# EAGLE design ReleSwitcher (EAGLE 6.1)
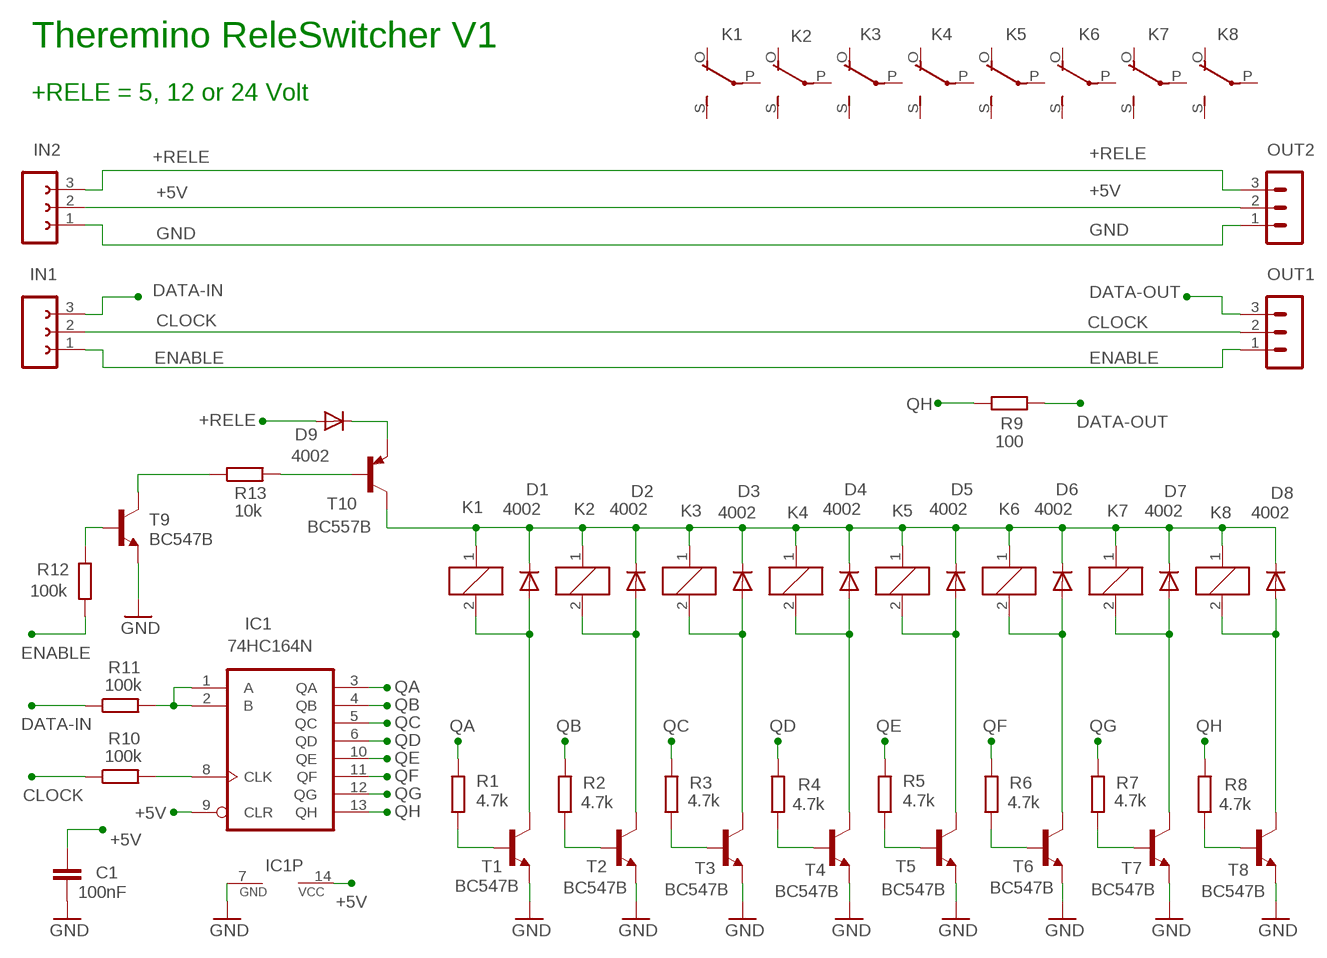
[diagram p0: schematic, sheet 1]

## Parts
C1  100nF  C-EU025-024X044  [C025-024X044]
D1  4002  DIODE-DO34-7  [DO34-7]
D2  4002  DIODE-DO34-7  [DO34-7]
D3  4002  DIODE-DO34-7  [DO34-7]
D4  4002  DIODE-DO34-7  [DO34-7]
D5  4002  DIODE-DO34-7  [DO34-7]
D6  4002  DIODE-DO34-7  [DO34-7]
D7  4002  DIODE-DO34-7  [DO34-7]
D8  4002  DIODE-DO34-7  [DO34-7]
D9  4002  DIODE-DO34-7  [DO34-7]
IC1  74HC164N  [DIL14]
IN1  FE03-1"  [FE03-1]
IN2  FE03-1"  [FE03-1]
K1  E3206S  [E3206S]
K2  E3206S  [E3206S]
K3  E3206S  [E3206S]
K4  E3206S  [E3206S]
K5  E3206S  [E3206S]
K6  E3206S  [E3206S]
K7  E3206S  [E3206S]
K8  E3206S  [E3206S]
OUT1  MA03-1N  [MA03-1]
OUT2  MA03-1N  [MA03-1]
R1  4.7k  R-EU_0204/7  [0204/7]
R2  4.7k  R-EU_0204/7  [0204/7]
R3  4.7k  R-EU_0204/7  [0204/7]
R4  4.7k  R-EU_0204/7  [0204/7]
R5  4.7k  R-EU_0207/10  [0207/10]
R6  4.7k  R-EU_0207/10  [0207/10]
R7  4.7k  R-EU_0207/10  [0207/10]
R8  4.7k  R-EU_0207/10  [0207/10]
R9  100  R-EU_0207/10  [0207/10]
R10  100k  R-EU_0207/15  [0207/15]
R11  100k  R-EU_0207/12  [0207/12]
R12  100k  R-EU_0207/15  [0207/15]
R13  10k  R-EU_0204/7  [0204/7]
T1  BC547B  -NPN-TO92-CBE  [TO92-CBE]
T2  BC547B  -NPN-TO92-CBE  [TO92-CBE]
T3  BC547B  -NPN-TO92-CBE  [TO92-CBE]
T4  BC547B  -NPN-TO92-CBE  [TO92-CBE]
T5  BC547B  -NPN-TO92-CBE  [TO92-CBE]
T6  BC547B  -NPN-TO92-CBE  [TO92-CBE]
T7  BC547B  -NPN-TO92-CBE  [TO92-CBE]
T8  BC547B  -NPN-TO92-CBE  [TO92-CBE]
T9  BC547B  -NPN-TO92-CBE  [TO92-CBE]
T10  BC557B  -PNP-TO92-CBE  [TO92-CBE]

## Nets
+5V: C1.1 IC1.9(CLR) IC1.14(VCC) IN2.2 OUT2.2
+RELE: D9.A IN2.3 OUT2.3
CLOCK: IN1.2 OUT1.2 R10.1
DATA-IN: IN1.3 R11.1
DATA-OUT: OUT1.3 R9.1
ENABLE: IN1.1 OUT1.1 R12.2
GND: C1.2 IC1.7(GND) IN2.1 OUT2.1 T1.E T2.E T3.E T4.E T5.E T6.E T7.E T8.E T9.E
N$1: R4.1 T4.B
N$2: R8.1 T8.B
N$4: R3.1 T3.B
N$5: D1.C D2.C D3.C D4.C D5.C D6.C D7.C D8.C K1.1 K2.1 K3.1 K4.1 K5.1 K6.1 K7.1 K8.1 T10.C
N$6: R2.1 T2.B
N$8: R1.1 T1.B
N$10: D4.A K4.2 T4.C
N$11: D3.A K3.2 T3.C
N$12: D2.A K2.2 T2.C
N$13: D1.A K1.2 T1.C
N$14: R13.1 T9.C
N$15: R13.2 T10.B
N$16: R12.1 T9.B
N$17: IC1.1(A) IC1.2(B) R11.2
N$18: IC1.8(CLK) R10.2
N$19: R7.1 T7.B
N$20: D9.C T10.E
N$22: R6.1 T6.B
N$25: R5.1 T5.B
N$27: D8.A K8.2 T8.C
N$28: D7.A K7.2 T7.C
N$29: D6.A K6.2 T6.C
N$30: D5.A K5.2 T5.C
QA: IC1.3(QA) R1.2
QB: IC1.4(QB) R2.2
QC: IC1.5(QC) R3.2
QD: IC1.6(QD) R4.2
QE: IC1.10(QE) R5.2
QF: IC1.11(QF) R6.2
QG: IC1.12(QG) R7.2
QH: IC1.13(QH) R8.2 R9.2
Unconnected: K1.O(2:O) K1.P(2:P) K1.S(2:S) K2.O(2:O) K2.P(2:P) K2.S(2:S) K3.O(2:O) K3.P(2:P) K3.S(2:S) K4.O(2:O) K4.P(2:P) K4.S(2:S) K5.O(2:O) K5.P(2:P) K5.S(2:S) K6.O(2:O) K6.P(2:P) K6.S(2:S) K7.O(2:O) K7.P(2:P) K7.S(2:S) K8.O(2:O) K8.P(2:P) K8.S(2:S)

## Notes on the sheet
- Theremino ReleSwitcher V1
- +RELE = 5, 12 or 24 Volt

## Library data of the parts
C1 = 00-LIVIO:C-EU: CAPACITOR, European symbol
D1-D9 = 00-LIVIO:DIODE-: DIODE
IC1 = 74xx-eu:74*164: 8-bit parallel out SHIFT REGISTER
IN1 IN2 = 02-con-lsta-F:FE03-1: FEMALE HEADER
K1-K8 = relay:E3206S: RELAY 1 x switch, Eichhoff/distributor Schukat
OUT1 OUT2 = 03-con-lstb-M:MA03-1: PIN HEADER
R1-R13 = 00-LIVIO:R-EU_: RESISTOR, European symbol
T1-T9 = 00-LIVIO:*-NPN-: NPN Transistror
T10 = 00-LIVIO:*-PNP-: PNP Transistror

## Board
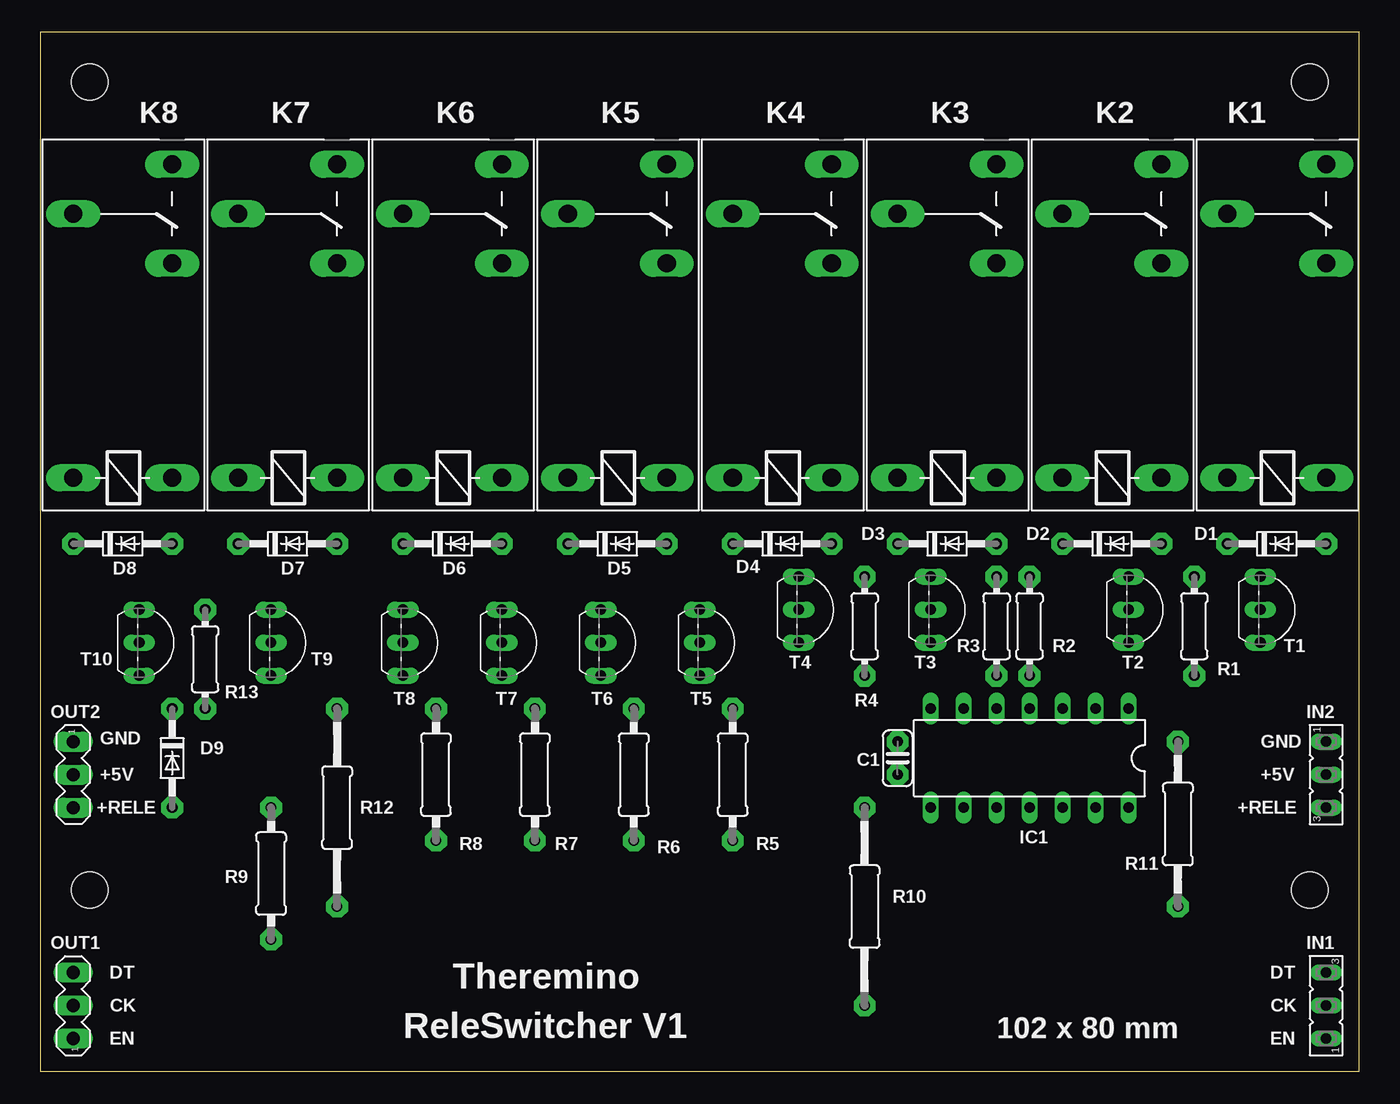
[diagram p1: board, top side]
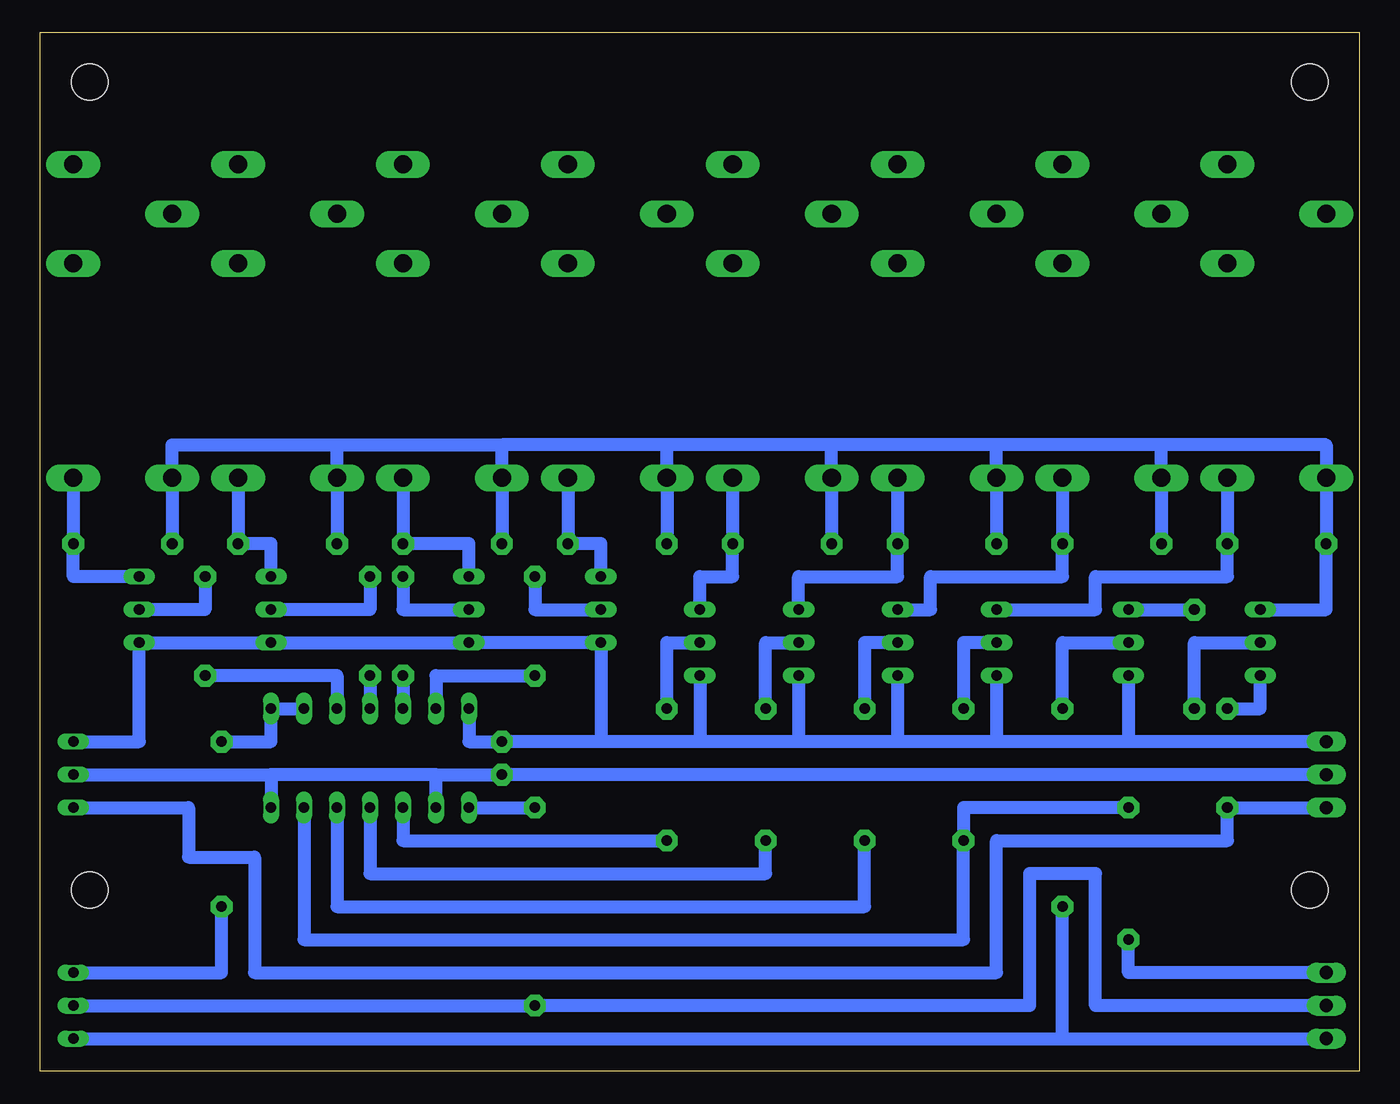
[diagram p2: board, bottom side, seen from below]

Size 101.6 x 80.01 mm. Coordinates in mm from the lower left corner, seen from the top.
Outline: 101.6,80.01 0,80.01 0,0 101.6,0 101.6,80.01
Copper layers (1*16): Top 0.035mm / dielectric 1.5mm / Bottom 0.035mm
Design rules: minimum track width 10mil, minimum drill 31mil, track to track 31mil, track to pad 31mil, pad to pad 31mil, via to via 31mil, smd to smd 31mil, copper to edge 31mil, drill to drill 8mil, minimum pad ring 5mil, minimum via ring 8mil, stop-mask expansion 4mil, vias tented up to drill 0mil, thermal gap 47mil
Holes 2.8 mm at 97.79,76.2 3.81,76.2 3.81,13.97 97.79,13.97

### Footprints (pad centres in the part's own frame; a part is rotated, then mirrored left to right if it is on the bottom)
C025-024X044 = drill 0.813 pad 1.676 octagon: 1 -1.27,0; 2 1.27,0
DO34-7 = drill 0.813 pad 1.676 octagon: A 3.81,0; C -3.81,0
DIL14 = drill 0.813 long: 1 -7.62,-3.81; 2 -5.08,-3.81; 3 -2.54,-3.81; 4 0,-3.81; 5 2.54,-3.81; 6 5.08,-3.81; 7 7.62,-3.81; 8 7.62,3.81; 9 5.08,3.81; 10 2.54,3.81; 11 0,3.81; 12 -2.54,3.81; 13 -5.08,3.81; 14 -7.62,3.81
FE03-1 = drill 0.813 long: 1 -2.54,0; 2 0,0; 3 2.54,0
E3206S = drill 1.397 long: 1 -3.175,3.81; 2 -3.175,-3.81; O 13.335,-3.81; P 17.145,3.81; S 20.955,-3.81
MA03-1 = drill 1.016 long: 1 -2.54,0; 2 0,0; 3 2.54,0
0204/7 = drill 0.813 pad 1.676 octagon: 1 -3.81,0; 2 3.81,0
0207/10 = drill 0.813 pad 1.676 octagon: 1 -5.08,0; 2 5.08,0
0207/15 = drill 0.813 pad 1.676 octagon: 1 -7.62,0; 2 7.62,0
0207/12 = drill 0.813 pad 1.676 octagon: 1 -6.35,0; 2 6.35,0
TO92-CBE = drill 0.813 long: B 0,0; C -2.54,0; E 2.54,0

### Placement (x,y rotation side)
C1  66.04,24.13 90 top
D1  95.25,40.64 0 top
D2  82.55,40.64 0 top
D3  69.85,40.64 0 top
D4  57.15,40.64 0 top
D5  44.45,40.64 0 top
D6  31.75,40.64 0 top
D7  19.05,40.64 0 top
D8  6.35,40.64 0 top
D9  10.16,24.13 270 top
IC1  76.2,24.13 180 top
IN1  99.06,5.08 90 top
IN2  99.06,22.86 270 top
K1  95.25,48.9 90 top
K2  82.55,48.9 90 top
K3  69.85,48.9 90 top
K4  57.15,48.9 90 top
K5  44.45,48.9 90 top
K6  31.75,48.9 90 top
K7  19.05,48.9 90 top
K8  6.35,48.9 90 top
OUT1  2.54,5.08 90 top
OUT2  2.54,22.86 270 top
R1  88.9,34.29 270 top
R2  76.2,34.29 270 top
R3  73.66,34.29 270 top
R4  63.5,34.29 270 top
R5  53.34,22.86 270 top
R6  45.72,22.86 270 top
R7  38.1,22.86 270 top
R8  30.48,22.86 270 top
R9  17.78,15.24 90 top
R10  63.5,12.7 90 top
R11  87.63,19.05 90 top
R12  22.86,20.32 270 top
R13  12.7,31.75 270 top
T1  93.98,35.56 270 top
T2  83.82,35.56 270 top
T3  68.58,35.56 270 top
T4  58.42,35.56 270 top
T5  50.8,33.02 270 top
T6  43.18,33.02 270 top
T7  35.56,33.02 270 top
T8  27.94,33.02 270 top
T9  17.78,33.02 270 top
T10  7.62,33.02 270 top

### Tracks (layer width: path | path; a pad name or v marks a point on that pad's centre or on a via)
+5V
  Bottom 1.016: IC1.9 71.12,22.86 | 71.12,22.86 83.82,22.86 | 83.82,22.86 IC1.14 | 71.12,22.86 C1.1 OUT2.2 | IN2.2 83.82,22.86
+RELE
  Bottom 1.016: IN2.3 90.17,20.32 90.17,16.51 85.09,16.51 85.09,7.62 27.94,7.62 27.94,17.78 10.16,17.78 D9.A OUT2.3
CLOCK
  Bottom 1.016: OUT1.2 20.32,5.08 20.32,15.24 25.4,15.24 25.4,5.08 R10.1 IN1.2
DATA-IN
  Bottom 1.016: IN1.3 87.63,7.62 R11.1
DATA-OUT
  Bottom 1.016: OUT1.3 17.78,7.62 R9.1
ENABLE
  Bottom 1.016: IN1.1 22.86,2.54 | 22.86,2.54 OUT1.1 | 22.86,2.54 R12.2
GND
  Bottom 1.016: IC1.7 68.58,25.4 C1.2 58.42,25.4 | 58.42,25.4 T4.E T3.E T2.E T1.E 93.98,25.4 IN2.1 | 27.94,25.4 35.56,25.4 | 35.56,25.4 43.18,25.4 | 43.18,25.4 50.8,25.4 | 50.8,25.4 58.42,25.4 | T6.E 43.18,25.4 | T5.E 50.8,25.4 | T7.E 35.56,25.4 | T8.E 27.94,25.4 | OUT2.1 17.78,25.4 | 17.78,25.4 27.94,25.4 | T9.E 17.78,25.4
N$1
  Bottom 1.016: R4.1 63.5,35.56 T4.B
N$2
  Bottom 1.016: T8.B 30.48,33.02 R8.1
N$4
  Bottom 1.016: R3.1 73.66,35.56 T3.B
N$5
  Bottom 1.016: D1.C K1.1 91.44,48.26 78.74,48.26 | 15.24,48.26 2.54,48.26 K8.1 D8.C 2.54,35.56 T10.C | 15.24,48.26 27.94,48.26 | 27.94,48.26 40.64,48.26 | 40.64,48.26 53.34,48.26 | 53.34,48.26 66.04,48.26 | 78.74,48.26 K2.1 D2.C | 78.74,48.26 66.04,48.26 | D3.C K3.1 66.04,48.26 | D4.C K4.1 53.34,48.26 | 15.24,48.26 K7.1 D7.C | 27.94,48.26 K6.1 D6.C | 40.64,48.26 K5.1 D5.C
N$6
  Bottom 1.016: R2.1 76.2,35.56 T2.B
N$8
  Bottom 1.016: R1.1 88.9,35.56 T1.B
N$10
  Bottom 1.016: K4.2 D4.A 58.42,40.64 T4.C
N$11
  Bottom 1.016: K3.2 D3.A 68.58,40.64 T3.C
N$12
  Bottom 1.016: K2.2 D2.A 83.82,40.64 T2.C
N$13
  Bottom 1.016: K1.2 D1.A 99.06,38.1 T1.C
N$14
  Bottom 1.016: T9.C R13.1
N$15
  Bottom 1.016: R13.2 12.7,33.02 T10.B
N$16
  Bottom 1.016: R12.1 22.86,33.02 T9.B
N$17
  Bottom 1.016: IC1.2 IC1.1 83.82,25.4 R11.2
N$18
  Bottom 1.016: IC1.8 R10.2
N$19
  Bottom 1.016: T7.B 38.1,33.02 R7.1
N$20
  Bottom 1.016: D9.C 7.62,27.94 T10.E
N$22
  Bottom 1.016: R6.1 45.72,33.02 T6.B
N$25
  Bottom 1.016: R5.1 53.34,33.02 T5.B
N$27
  Bottom 1.016: K8.2 D8.A 10.16,38.1 20.32,38.1 20.32,35.56 T8.C
N$28
  Bottom 1.016: K7.2 D7.A 22.86,38.1 33.02,38.1 33.02,35.56 T7.C
N$29
  Bottom 1.016: K6.2 D6.A 35.56,38.1 43.18,38.1 T6.C
N$30
  Bottom 1.016: K5.2 D5.A 48.26,38.1 50.8,38.1 T5.C
QA
  Bottom 1.016: R1.2 78.74,30.48 IC1.3
QB
  Bottom 1.016: R2.2 IC1.4
QC
  Bottom 1.016: R3.2 IC1.5
QD
  Bottom 1.016: R4.2 71.12,30.48 IC1.6
QE
  Bottom 1.016: IC1.10 73.66,17.78 R5.2
QF
  Bottom 1.016: IC1.11 76.2,15.24 45.72,15.24 R6.2
QG
  Bottom 1.016: IC1.12 78.74,12.7 38.1,12.7 R7.2
QH
  Bottom 1.016: IC1.13 81.28,10.16 30.48,10.16 R8.2 30.48,20.32 R9.2

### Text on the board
tNames: GND | GND | +5V | +5V | +RELE | +RELE | DT | DT | Theremino | CK | CK | ReleSwitcher V1 | 102 x 80 mm | EN | EN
